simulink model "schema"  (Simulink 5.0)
settings: Solver=ode4  StartTime=0  StopTime=cas_simulacie  FixedStep=krok  RelTol=1e-3
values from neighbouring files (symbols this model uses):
  D = uicontrol(gcf,   'Style','edit',   'ForegroundColor','black',   'BackgroundColor',[1 1 1],   'String',num2str(D),   'Position',[100 105 80 20],   'CallBack',['D=str2num(get(D,''String''));'])    [id_system.m]    (also in param.m = D1; param2.m = D2)
  T = uicontrol(gcf,   'Style','edit',   'ForegroundColor','black',   'BackgroundColor',[1 1 1],   'String',num2str(T),   'Position',[100 80 80 20],    'CallBack',['T=str2num(get(T,''String''));'])    [id_system.m]    (also in param.m = T1; param2.m = T2)
  t0 = uicontrol(gcf,   'Style','edit',   'ForegroundColor','black',   'BackgroundColor',[1 1 1],   'String',num2str(t0),   'Position',[100 305 80 20],   'CallBack',['t0=str2num(get(t0,''String''));'])    [id_system.m]    (also in sus1.m = uicontrol(gcf,   'Style','edit',   'ForegroundColor','black'; sus2.m = uicontrol(gcf,   'Style','edit',   'ForegroundColor','black')
  u_0 = uicontrol(gcf,   'Style','edit',   'ForegroundColor','black',   'BackgroundColor',[1 1 1],   'String',num2str(u_0),   'Position',[100 230 80 20],   'CallBack',['u_0=str2num(get(u_0,''String''));'])    [id_system.m]    (also in sus1.m = uicontrol(gcf,   'Style','edit',   'ForegroundColor','black'; sus2.m = uicontrol(gcf,   'Style','edit',   'ForegroundColor','black')
  u_nek = uicontrol(gcf,   'Style','edit',   'ForegroundColor','black',   'BackgroundColor',[1 1 1],   'String',num2str(u_nek),   'Position',[100 205 80 20],   'CallBack',['u_nek=str2num(get(u_nek,''String''));'])    [id_system.m]    (also in sus1.m = uicontrol(gcf,   'Style','edit',   'ForegroundColor','black'; sus2.m = uicontrol(gcf,   'Style','edit',   'ForegroundColor','black')
  y_0 = uicontrol(gcf,   'Style','edit',   'ForegroundColor','black',   'BackgroundColor',[1 1 1],   'String', num2str(y_0),   'Position',[100 180 80 20],   'CallBack',['y_0=str2num(get(y_0,''String''));'])    [id_system.m]    (also in sus1.m = uicontrol(gcf,   'Style','edit',   'ForegroundColor','black'; sus2.m = uicontrol(gcf,   'Style','edit',   'ForegroundColor','black')
  Z = uicontrol(gcf,   'Style','edit',   'ForegroundColor','black',   'BackgroundColor',[1 1 1],   'String',num2str(Z) ,   'Position',[100 130 80 18],   'CallBack',['Z=str2num(get(Z,''String''));'])    [id_system.m]    (also in param.m = Z1; param2.m = Z2)

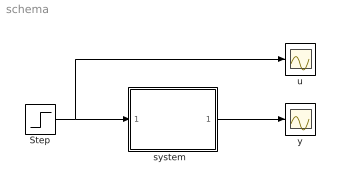
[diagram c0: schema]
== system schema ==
  Step : Step  Time=t0  Before=u_0  After=u_nek  SampleTime=0
  "system  " : Subsystem
  u : Scope
  y : Scope
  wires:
  Step/1 -> u/1, "system  "/1(In1)
  "system  "/1(Out1) -> y/1

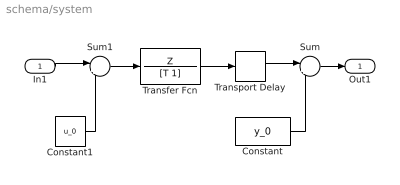
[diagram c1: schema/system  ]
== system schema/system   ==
  In1 : Inport
  Constant : Constant  Value=y_0
  Constant1 : Constant  Value=u_0
  Sum : Sum  Inputs=|++
  Sum1 : Sum  Inputs=|+-
  Transfer Fcn : TransferFcn  Numerator=Z  Denominator=[T 1]
  Transport Delay : TransportDelay  DelayTime=D
  Out1 : Outport
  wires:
  Transfer Fcn/1 -> Transport Delay/1
  Transport Delay/1 -> Sum/1
  Constant/1 -> Sum/2
  Sum1/1 -> Transfer Fcn/1
  Constant1/1 -> Sum1/2
  In1/1 -> Sum1/1
  Sum/1 -> Out1/1
